FUNCTION FC 69 : VOID
TITLE =BLOCK FOR CLAMPS
AUTHOR : Esposito
FAMILY : EGAL_srl
NAME : CLAMPS
VERSION : 0.1

BEGIN
NETWORK
TITLE =CONDITIONS FOR START CLAMPS CIRCUIT
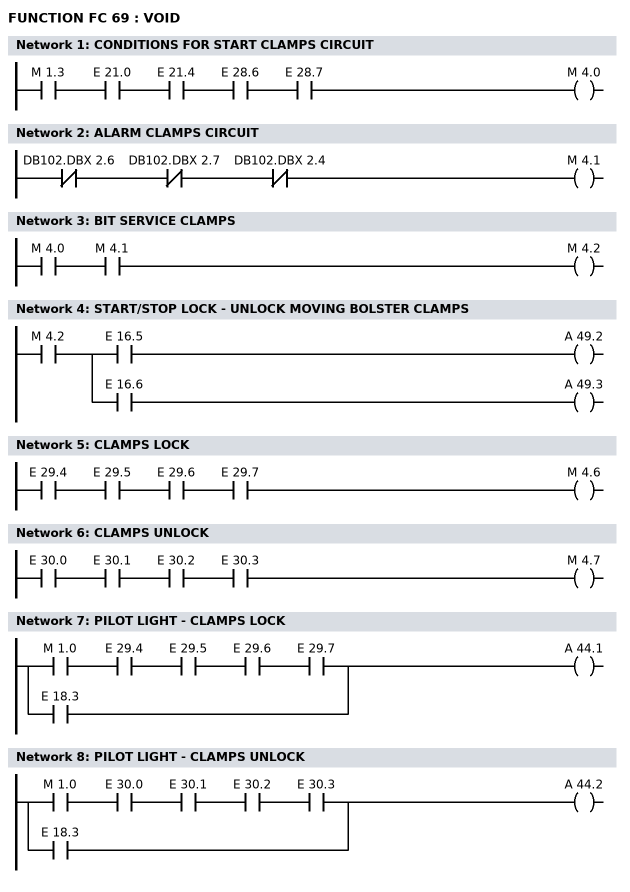
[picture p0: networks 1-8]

      U     M      1.3;
      U     E     21.0;
      U     E     21.4;
      U     E     28.6;
      U     E     28.7;
      =     M      4.0;
NETWORK
TITLE =ALARM CLAMPS CIRCUIT

      UN    DB102.DBX    2.6;
      UN    DB102.DBX    2.7;
      UN    DB102.DBX    2.4;
      =     M      4.1;
NETWORK
TITLE =BIT SERVICE CLAMPS

      U     M      4.0;
      U     M      4.1;
      =     M      4.2;
NETWORK
TITLE =START/STOP LOCK - UNLOCK MOVING BOLSTER CLAMPS

      U     M      4.2;
      =     L      0.0;
      U     L      0.0;
      U     E     16.5;
      =     A     49.2;
      U     L      0.0;
      U     E     16.6;
      =     A     49.3;
NETWORK
TITLE =CLAMPS LOCK

      U     E     29.4;
      U     E     29.5;
      U     E     29.6;
      U     E     29.7;
      =     M      4.6;
NETWORK
TITLE =CLAMPS UNLOCK

      U     E     30.0;
      U     E     30.1;
      U     E     30.2;
      U     E     30.3;
      =     M      4.7;
NETWORK
TITLE =PILOT LIGHT - CLAMPS LOCK

      U     M      1.0;
      U     E     29.4;
      U     E     29.5;
      U     E     29.6;
      U     E     29.7;
      O     E     18.3;
      =     A     44.1;
NETWORK
TITLE =PILOT LIGHT - CLAMPS UNLOCK

      U     M      1.0;
      U     E     30.0;
      U     E     30.1;
      U     E     30.2;
      U     E     30.3;
      O     E     18.3;
      =     A     44.2;
END_FUNCTION

